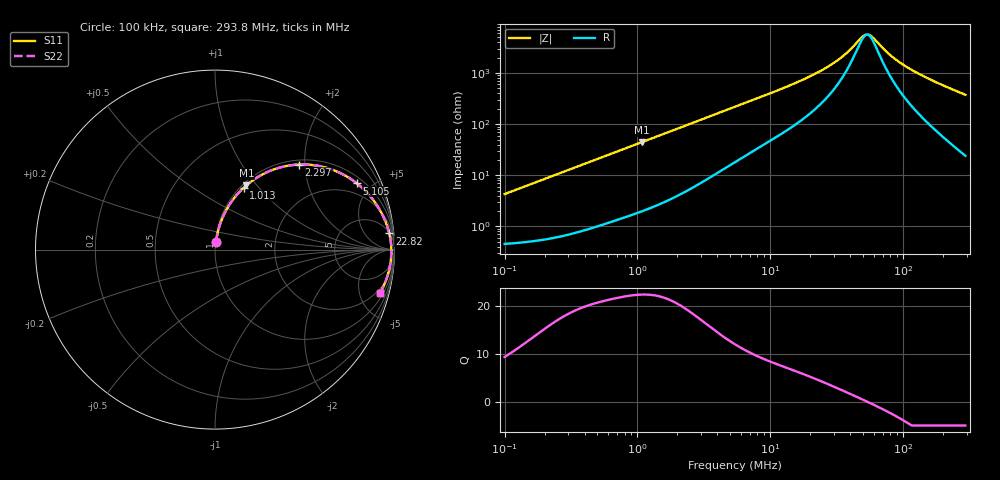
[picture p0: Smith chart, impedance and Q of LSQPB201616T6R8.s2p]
! LSQPB201616T6R8  S-PARAMETER MODEL  ( General Type )
! Model Generated by TAIYO YUDEN Corporation (http://www.ty-top.com)
! Version 2.0
! TAIYO YUDEN Control No. 100810NC14SB-FKC
! Copyright(c) 2008 TAIYO YUDEN CO.,LTD. All Rights Reserved.
! Product Description (link to TY-COMPAS)
! https://ds.yuden.co.jp/TYCOMPAS/or/detail?pn=LSQPB201616T6R8M&u=M
! Products Name : Inductors
! Characteristics :
!  Inductance : 6.8 uH , SRF(min) : 39 MHz , DC Resistance(max) : 0.429 Ohm
!  Rated Current : Saturation :550 mA , Temp Rise : 560 mA (40 degC)
!  Case Size : 2.0 x 1.6 / 0.079 x 0.063 [mm/inch] , Thickness : 1.6 / 0.063 [mm/inch]
!  (Conditions: Temperature = 25 degC , DC Bias Current/Voltage = 0A / 0V)
! External Node Assignments :
!  1  o---GGG---o  2
! GND o---------o GND
! Frequency Range : 0.1MHz  -  293.796821MHz  [ 402 STEP ]
# MHz S RI R 50
! Freq[MHz].  S11 Real  S11 Imag  S21 Real  S21 Imag  S12 Real  S12 Imag  S22 Real  S22 Imag
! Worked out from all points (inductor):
!   401 points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, 100 kHz to 293.8 MHz, reference 50 ohm
!   read as one part in series: L = 6.77 uH near 104.1 kHz
!   highest Q = 22.5 at 1.076 MHz (marker M1), where L = 6.55 uH
!   self-resonance near 53.5 MHz
!   S11 on the Smith chart (normalised r, x): 100 kHz: 1.01, +0.09; 1.013 MHz: 1.04, +0.83; 2.297 MHz: 1.10, +1.87; 5.105 MHz: 1.33, +4.10; 22.82 MHz: 5, +20; 293.8 MHz: 1.48, -7.49
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0.1  0.00633 0.0422  0.9937 -0.0422  0.9937 -0.0422  0.00633 0.0422
0.380976  0.0324 0.1535  0.9676 -0.1535  0.9676 -0.1535  0.0324 0.1535
0.653117  0.0785 0.2468  0.9215 -0.2468  0.9215 -0.2468  0.0785 0.2468
1.01329  0.1593 0.3443  0.8407 -0.3443  0.8407 -0.3443  0.1593 0.3443
1.075831  0.1747 0.3581  0.8253 -0.3581  0.8253 -0.3581  0.1747 0.3581
1.451429  0.2705 0.4222  0.7295 -0.4222  0.7295 -0.4222  0.2705 0.4222
2.297251  0.4687 0.4741  0.5313 -0.4741  0.5313 -0.4741  0.4687 0.4741
3.290566  0.6328 0.4523  0.3672 -0.4523  0.3672 -0.4523  0.6328 0.4523
5.105205  0.7907 0.3688  0.2093 -0.3688  0.2093 -0.3688  0.7907 0.3688
5.420303  0.8072 0.3551  0.1928 -0.3551  0.1928 -0.3551  0.8072 0.3551
9.670679  0.9144 0.2274  0.0856 -0.2274  0.0856 -0.2274  0.9144 0.2274
20.65007  0.968 0.1029  0.032 -0.1029  0.032 -0.1029  0.968 0.1029
22.81771  0.9713 0.0901  0.0287 -0.0901  0.0287 -0.0901  0.9713 0.0901
33.34297  0.9793 0.0469  0.0207 -0.0469  0.0207 -0.0469  0.9793 0.0469
39.11697  0.9811 0.0306  0.0189 -0.0306  0.0189 -0.0306  0.9811 0.0306
48.72328  0.9824 0.00902  0.0176 -0.00902  0.0176 -0.00902  0.9824 0.00902
52.77363  0.9827 0.00132  0.0173 -0.00132  0.0173 -0.00132  0.9827 0.00132
58.31329  0.9827 -0.00832  0.0173 0.00832  0.0173 0.00832  0.9827 -0.00832
78.67184  0.9816 -0.0381  0.0184 0.0381  0.0184 0.0381  0.9816 -0.0381
97.992  0.9793 -0.0619  0.0207 0.0619  0.0207 0.0619  0.9793 -0.0619
132.2033  0.9732 -0.099  0.0268 0.099  0.0268 0.099  0.9732 -0.099
293.7968  0.9203 -0.2406  0.0797 0.2406  0.0797 0.2406  0.9203 -0.2406
